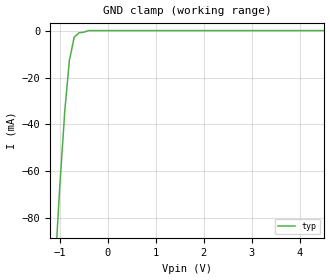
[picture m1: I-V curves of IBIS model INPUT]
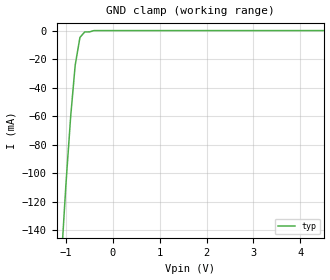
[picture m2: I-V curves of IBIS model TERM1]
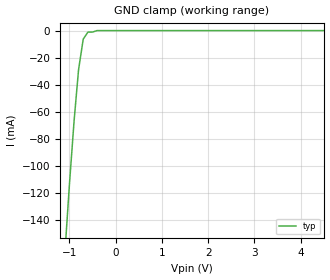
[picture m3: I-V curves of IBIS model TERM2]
|   PERICOM SEMICONDUCTOR CORP
|   IBIS Model of PI5A3157
|   Product Family: 5A
|   SC70 (C) Package
[IBIS Ver] 3.2
[Comment char] |_char
[File Name] pi5a3157b_c_33v.ibs
[File Rev] 2.1
[Source] File originated at Pericom Semiconductor Corp.
[Date] 07/28/17
[Disclaimer] (C) Copyright PERICOM Semiconductor Corporation
   All rights reserved
  Pericom Semiconductor Corporation hereby grants the user of
  this IBIS model a non-exclusive, nontransferable license to
  use this IBIS model under the following terms.
  This IBIS model is provided on an "AS IS" basis and Pericom
  makes absolutely no warranty with respect to the information
  contained herein. PERICOM DISCLAIMS AND CUSTOMER WAIVES ALL
  WARRANTIES, EXPRESSED OR IMPLIED, INCLUDING WARRANTIES OF
  MERCHANTABILITY OR FITNESS FOR A PARTICULAR PURPOSE. The
  entire risk as to quality and performance is with the customer.
  Accordingly, in no event shall the company be liable for any
  damages, whether in contract or tort, including any lost
  profits or other incidental, consequential, exemplary, or
  punitive damages arising out of the use or application of the
  IBIS model provided in this package. Further, Pericom reserves
  the right to make changes without notice to any product herein
  to improve reliability, function, or design. Pericom does not
  convey any license under patent rights or any other intellectual
  property rights, including those of third parties.
  The user is granted this license only to use the IBIS model
  and is not granted rights to sell, load, rent, lease or license
  the IBIS model in whole or in part, or in modified form to anyone
  other than user. User may modify the IBIS model to suit its specific
  application but rights to derivative works and such modifications
  shall belong to Pericom.
  Pericom is not obligated to provide maintenance or support
  for the licensed IBIS model.
  Contact Pericom at ATTN: APPLICATION ENGINEERING / IBIS MODELS
  1545 Barber Lane Milpitas, CA 95035 USA.
[Component] PI5A3157B
[Manufacturer] Pericom Semiconductor Corp.
[Package]
| variable   typ   min  max
R_pkg   0.04159ohm   NA   NA
L_pkg   0.97147nH   NA   NA
C_pkg   0.28606pF   NA   NA
[Pin] signal_name   model_name   R_pin   L_pin   C_pin
1   B1   TERM1   0.04441   1.10870nH   0.32525pF
2   GND   POWER   0.03657   0.79240nH   0.22999pF
3   B0   TERM1   0.04436   1.10760nH   0.32525pF
4   A   TERM2   0.04436   1.10760nH   0.32525pF
5   VCC   POWER   0.03657   0.79240nH   0.22999pF
6   S   INPUT   0.04441   1.10870nH   0.32525pF
[Series Switch Groups]
On 1 /
Off 2 /
[Series Pin Mapping]   pin_2   model_name  function_table_group
4   1   SWITCH1   1
4   3   SWITCH1   2
|   Model SWITCH1
[Model] SWITCH1
Model_type Series_switch
| variable   typ   min   max
C_comp   18.5000pF  NA   NA
[Voltage Range]   3.3000V   NA   NA
[POWER Clamp Reference]   3.3000V   NA   NA
[GND Clamp Reference]   0.0000V   NA   NA
[On]
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[OFF]
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| Models and submodels in the file (4): INPUT (Input), SWITCH1 (Series_switch), TERM1 (Terminator), TERM2 (Terminator)
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|   Model INPUT
[Model] INPUT
Model_type Input
Vinl = 825mV
Vinh = 2.310V
| variable   typ   min   max
C_comp   2.3000pF   NA   NA
[Voltage Range]   3.3000V   NA   NA
[GND Clamp Reference]   0.0000V   NA   NA
[POWER Clamp Reference]   3.3000V   NA   NA
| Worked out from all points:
|   GND clamp passes 1 mA (typ) near -0.60 V on its own axis
[GND Clamp]
| Voltage   I(typ)   I(min)   I(max)
-3.3V     -906.3mA   NA         NA
-1.1V     -101mA     NA         NA
-999.3mV  -65.49mA   NA         NA
-898.2mV  -34.4mA    NA         NA
-802mV    -12.71mA   NA         NA
-700.9mV  -2.78mA    NA         NA
-599.7mV  -950uA     NA         NA
-402.6mV  0A         NA         NA
6.602V    0A         NA         NA
[POWER Clamp]   |Note: Vtable = Vcc - Voutput
| Voltage   I(typ)   I(min)   I(max)
-3.3V     0A         NA         NA
0V        0A         NA         NA
|   Model TERM1
[Model] TERM1
Model_type Terminator
| variable   typ   min   max
C_comp   6.5000pF   NA   NA
[Voltage Range]   3.3000V   NA   NA
[GND Clamp Reference]   0.0000V   NA   NA
[POWER Clamp Reference]   3.3000V   NA   NA
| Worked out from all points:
|   GND clamp passes 1 mA (typ) near -0.60 V on its own axis
[GND Clamp]
| Voltage   I(typ)   I(min)  I(max)
-3.3V     -1.236A    NA         NA
-1.1V     -162.2mA   NA         NA
-999.3mV  -107.7mA   NA         NA
-898.2mV  -60.09mA   NA         NA
-802mV    -24.25mA   NA         NA
-700.8mV  -4.84mA    NA         NA
-599.7mV  -960uA     NA         NA
-498.4mV  -920uA     NA         NA
-402.6mV  0A         NA         NA
6.602V    0A         NA         NA
[POWER Clamp]   |Note: Vtable = Vcc - Voutput
| Voltage   I(typ)   I(min)   I(max)
-3.3V     0A         NA         NA
0V        0A         NA         NA
|   Model TERM2
[Model] TERM2
Model_type Terminator
| variable   typ   min   max
C_comp   11.5000pF   NA   NA
[Voltage Range]   3.3000V   NA   NA
[GND Clamp Reference]   0.0000V   NA   NA
[POWER Clamp Reference]   3.3000V   NA   NA
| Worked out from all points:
|   GND clamp passes 1 mA (typ) near -0.49 V on its own axis
[GND Clamp]
| Voltage   I(typ)   I(min)  I(max)
-3.3V     -1.118A    NA         NA
-1.1V     -165.5mA   NA         NA
-999.3mV  -113.4mA   NA         NA
-898.2mV  -66.37mA   NA         NA
-802mV    -28.86mA   NA         NA
-700.8mV  -6.27mA    NA         NA
-599.7mV  -1.13mA    NA         NA
-498.4mV  -1.09mA    NA         NA
-402.6mV  0A         NA         NA
6.602V    0A         NA         NA
[POWER Clamp]   |Note: Vtable = Vcc - Voutput
| Voltage   I(typ)   I(min)   I(max)
-3.3V     0A         NA         NA
0V        0A         NA         NA
